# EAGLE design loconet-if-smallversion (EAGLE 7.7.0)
Assembly variants: var1
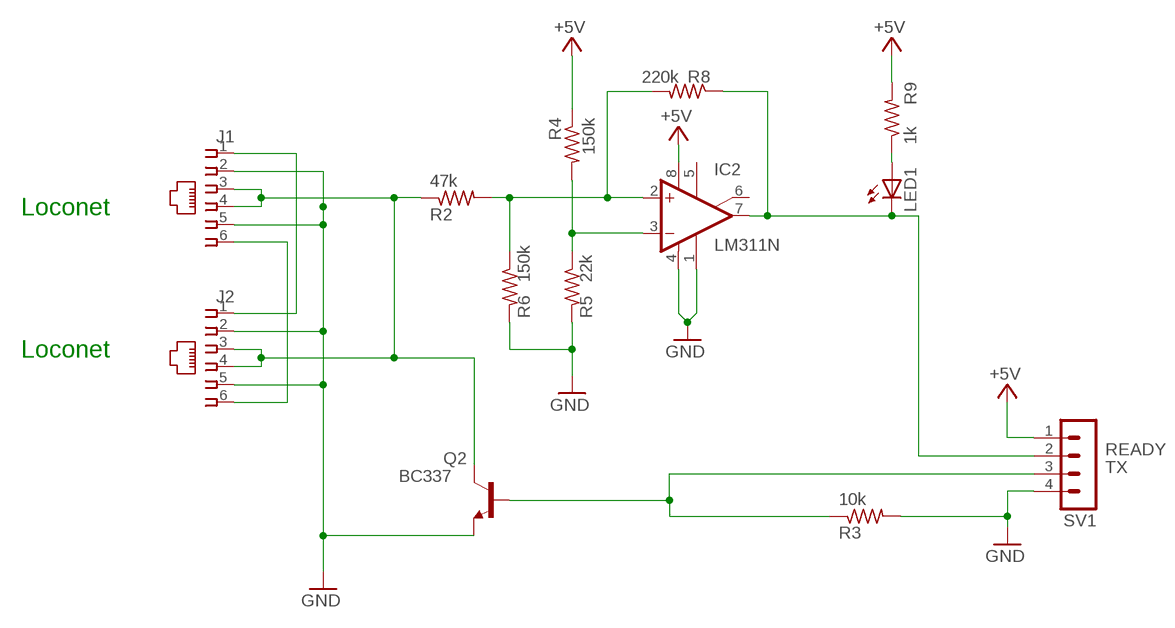
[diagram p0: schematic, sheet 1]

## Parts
IC2  LM311N  [DIL08]
J1  520425-3  [520425-3]
J2  520425-3  [520425-3]
LED1  LED3MM  [LED3MM]
Q2  BC337  2N3904  [TO92]
R2  47k  R-US_0204/7  [0204/7]
R3  10k  R-US_0204/7  [0204/7]
R4  150k  R-US_0204/7  [0204/7]
R5  22k  R-US_0204/7  [0204/7]
R6  150k  R-US_0204/7  [0204/7]
R8  220k  R-US_0204/7  [0204/7]
R9  1k  R-US_0204/7  [0204/7]
SV1  MA04-1  [MA04-1]

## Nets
+5V [power]: IC2.8(V+) R4.1 R9.2 SV1.1
GND: IC2.1(GND) IC2.4(V-) J1.2 J1.5 J2.2 J2.5 Q2.3(E) R3.2 R5.2 R6.2 SV1.4
N$1: LED1.A R9.1
N$6: J1.1 J2.1
N$10: J1.6 J2.6
N$14: IC2.2(+IN) R2.2 R6.1 R8.2
N$16: J1.3 J1.4 J2.3 J2.4 Q2.1(C) R2.1
N$17: IC2.3(-IN) R4.2 R5.1
READY: IC2.7(OUT) LED1.K(C) R8.1 SV1.2
TX: Q2.2(B) R3.1 SV1.3
Unconnected: IC2.5(ON) IC2.6(ON/STR)

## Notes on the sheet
- Loconet
- Loconet

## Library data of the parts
IC2 = linear:LM311: COMPARATOR
J1 J2 = con-amp:520425-3: AMP connector
LED1 = led:LED: LED
Q2 = transistor-npn:2N3904: NPN Transistor
R2-R6 R8 R9 = rcl:R-US_: RESISTOR, American symbol
SV1 = con-lstb:MA04-1: PIN HEADER; OC_FARNELL: unknown; OC_NEWARK: unknown

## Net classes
0 default: width 0.457 mm
1 power: width 1.016 mm

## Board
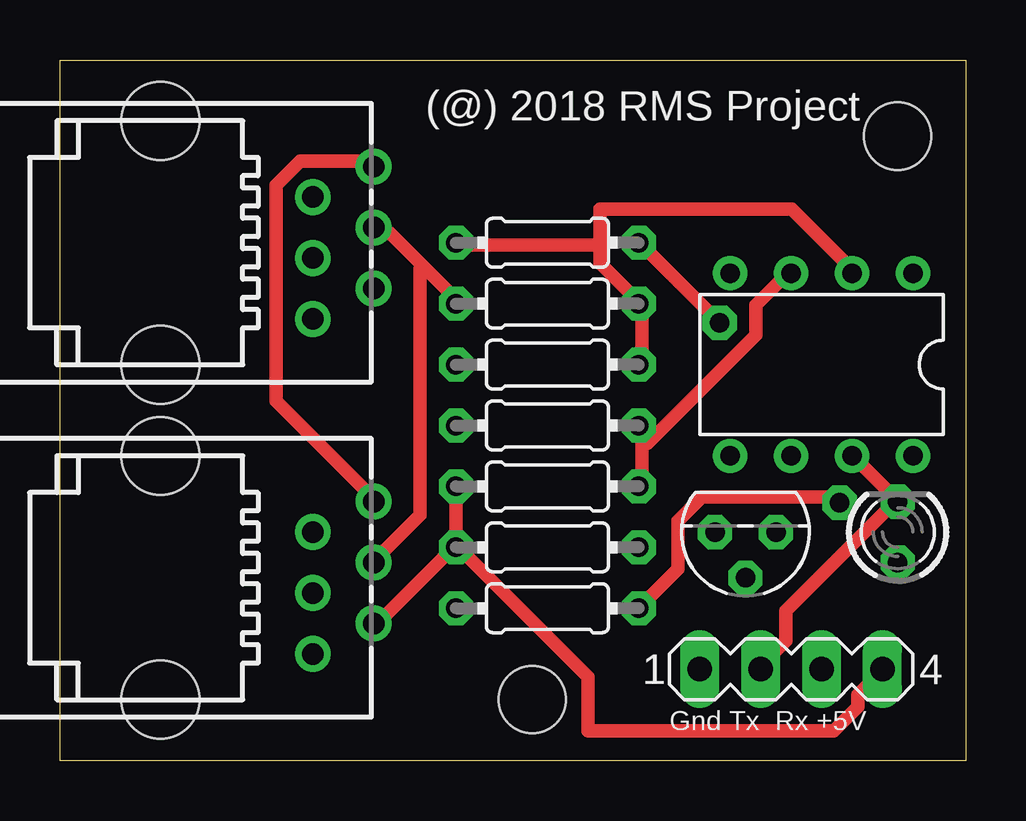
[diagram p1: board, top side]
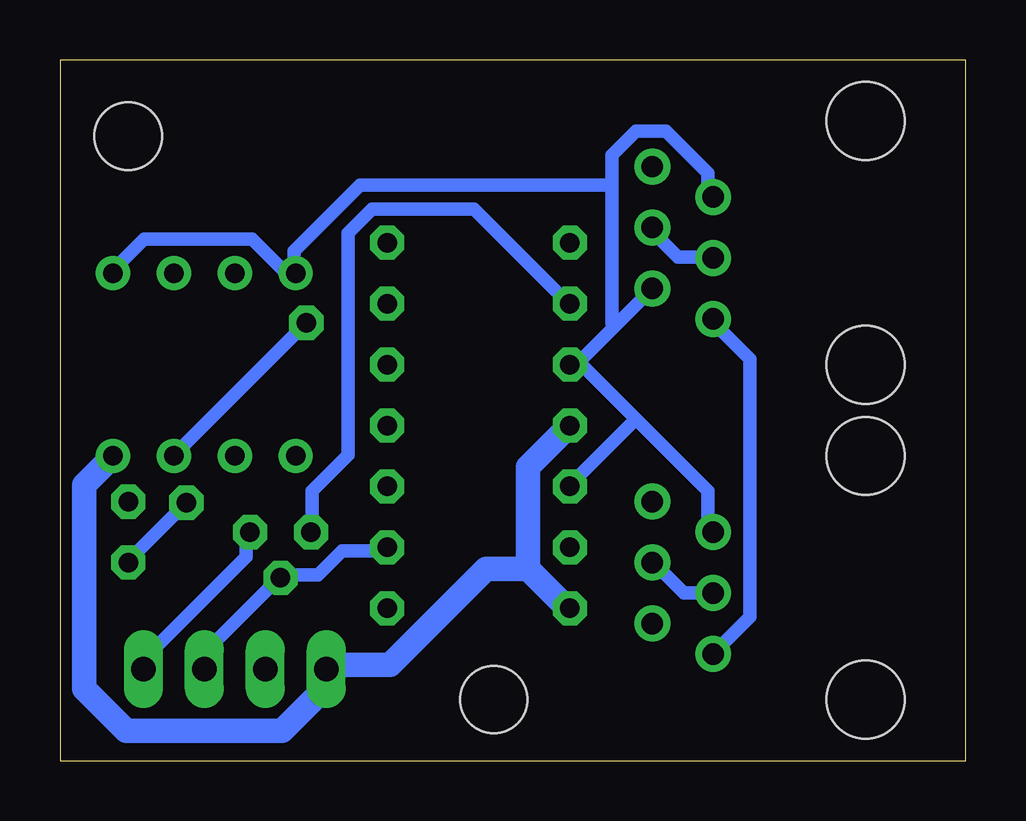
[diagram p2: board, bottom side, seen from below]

Size 37.77 x 29.22 mm. Coordinates in mm from the lower left corner, seen from the top.
Outline: 0,29.22 37.77,29.22 37.77,0 0,0 0,29.22
Copper layers (1*16): Top 0.02mm / dielectric 1.5mm / Bottom 0.02mm
Design rules "default *": minimum track width 22mil, minimum drill 32mil, track to track 16mil, track to pad 16mil, pad to pad 16mil, via to via 16mil, smd to smd 16mil, copper to edge 20mil, drill to drill 12mil, minimum pad ring 12mil, minimum via ring 12mil, stop-mask expansion 4mil, vias tented up to drill 0mil, thermal gap 10mil
Holes 2.8 mm at 19.68,2.55 34.92,26.05

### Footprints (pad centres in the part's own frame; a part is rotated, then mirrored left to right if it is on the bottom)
DIL08 = drill 0.813 pad 1.27: 1 -3.81,-3.81; 2 -1.27,-3.81; 3 1.27,-3.81; 4 3.81,-3.81; 5 3.81,3.81; 6 1.27,3.81; 7 -1.27,3.81; 8 -3.81,3.81
520425-3 = drill 0.889: 1 -3.175,8.001; 2 -1.905,5.461; 3 -0.635,8.001; 4 0.635,5.461; 5 1.905,8.001; 6 3.175,5.461 | hole 3.251: -5.08,-0.889; 5.08,-0.889
LED3MM = drill 0.813 octagon: A -1.27,0; K 1.27,0
TO92 = drill 0.813 octagon: 1 1.27,0; 2 0,1.905; 3 -1.27,0
0204/7 = drill 0.813 octagon: 1 -3.81,0; 2 3.81,0
MA04-1 = drill 1.016 long: 1 -3.81,0; 2 -1.27,0; 3 1.27,0; 4 3.81,0

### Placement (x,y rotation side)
IC2  31.75,16.52 180 top
J1  5.08,7.63 270 top
J2  5.08,21.6 270 top
LED1  34.92,9.54 90 top
Q2  28.57,9.54 180 top
R2  20.32,19.06 0 top
R3  20.32,8.9 180 top
R4  20.32,13.98 0 top
R5  20.32,11.44 180 top
R6  20.32,16.52 180 top
R8  20.32,21.6 180 top
R9  20.32,6.36 180 top
SV1  30.48,3.82 0 top

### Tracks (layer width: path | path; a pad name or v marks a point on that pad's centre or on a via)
+5V
  Bottom 1.016: 18.25,8.01 16.75,6.51 R9.2 | 18.25,8.01 18.25,12.26 16.75,13.76 R4.1 | IC2.8 35.75,12.51 36.75,11.51 36.75,3.01 35,1.26 28.5,1.26 26.75,3.01 26.75,3.76 SV1.1 26.25,4.01 24,4.01 20,8.01 18.25,8.01
GND
  Top 0.559: R3.2 16.5,9.01 16.5,11.26 R5.2 | J1.5 13.25,5.76 16.25,8.76 R3.2 | SV1.4 34.25,3.76 33.25,2.76 33.25,2.26 32.25,1.26 22,1.26 22,3.51 16.75,8.76 R3.2
  Bottom 0.559: Q2.3 30,9.51 30,8.51 34.5,4.01 SV1.4 | IC2.1 35.5,20.51 34.25,21.76 29.75,21.76 28.5,20.51 28,20.51 IC2.4 28,20.76 28,21.26 25.25,24.01 14.75,24.01 | 14.62,18.14 13.25,19.51 J2.5 | 14.62,18.14 16,16.76 16.5,16.76 R6.2 16,16.51 13.75,14.26 | 13.75,14.26 10.75,11.26 10.75,9.76 J1.2 | 14.75,24.01 14.75,18.26 14.62,18.14 | 14.75,24.01 14.75,25.26 13.75,26.26 12.5,26.26 10.75,24.51 10.75,23.51 J2.2 | 13.75,14.26 16.5,11.51 R5.2
N$1  (via drill 0.81)
  Top 0.559: v32.5,10.76 32.5,11.01 26.75,11.01 25.75,10.01 25.75,8.01 24.25,6.51 R9.1
  Bottom 0.559: v32.5,10.76 34.75,8.51 LED1.A
N$6
  Top 0.559: J1.1 13,11.01 9,15.01 9,24.01 10,25.01 13,25.01 J2.1
N$10
  Bottom 0.559: J1.6 10.5,4.51 9,6.01 9,16.76 10.5,18.26 J2.6
N$14
  Top 0.559: R6.1 24.25,16.76 24.25,19.01 R2.2 24,19.26 22.5,20.76 22.5,21.51 | 22.5,21.51 16.75,21.51 R8.2 | 22.5,21.51 22.5,23.01 30.5,23.01 33,20.51 IC2.2
N$16
  Top 0.559: 15.12,20.64 13.75,22.01 13.25,22.01 J2.3 | 15.12,20.64 16.5,19.26 R2.1 | J1.3 13.25,8.51 15,10.26 15,20.51 15.12,20.64
  Bottom 0.559: J1.4 10.75,7.01 11.75,7.01 13,8.26 J1.3 | Q2.1 27.25,9.76 27.25,11.26 25.75,12.76 25.75,22.01 24.75,23.01 20.5,23.01 16.75,19.26 R2.1 | J2.4 10.75,21.01 12,21.01 13,22.01 J2.3
N$17
  Top 0.559: 24.25,13.26 24.25,13.76 R4.2 | 24.25,13.26 24.25,11.51 R5.1 | IC2.3 30.25,20.26 29,19.01 29,17.76 24.5,13.26 24.25,13.26
READY  (via drill 0.81)
  Top 0.559: IC2.7 33.25,12.51 34.75,11.01 LED1.K 34.75,10.76 30.25,6.26 30.25,5.01 29.25,4.01 SV1.2 | v27.5,18.26 24.25,21.51 R8.1
  Bottom 0.559: v27.5,18.26 33,12.76 IC2.7
TX
  Bottom 0.559: R3.1 24.25,8.76 26,8.76 27,7.76 28.5,7.76 Q2.2 28.75,7.51 31.75,4.51 SV1.3

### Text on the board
tNames: (@) 2018 RMS Project | Gnd Tx Rx +5V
